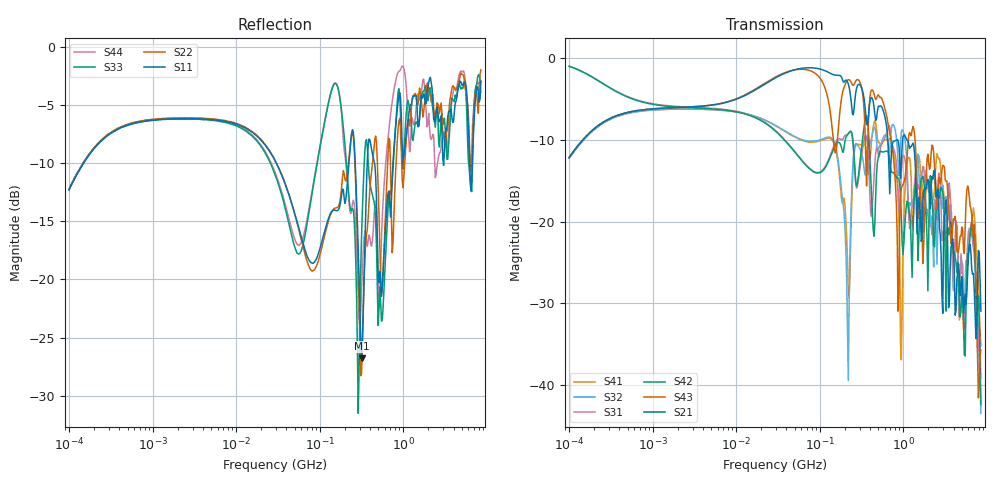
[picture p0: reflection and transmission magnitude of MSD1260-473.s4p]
# MHz S MA R 50
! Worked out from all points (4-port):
!   498 points, 100 kHz to 8.5 GHz, reference 50 ohm
!   strongest paths, dB at 100 kHz, 1.698 MHz, 29.49 MHz, 500.7 MHz, 8.5 GHz:
!     S21: -12.1, -6.1, -2.4, -6.0, -31.0
!     S43: -12.2, -6.1, -2.3, -4.5, -35.7
!     S42: -1.0, -5.9, -8.9, -12.2, -42.4
!     S31: -1.0, -5.9, -8.8, -11.6, -39.2
!     S32: -12.3, -6.2, -8.2, -11.3, -43.5
!     S41: -12.3, -6.2, -8.3, -10.3, -35.2
!   lowest |S11| = -26.8 dB at 317.1 MHz (marker M1), VSWR 1.10, Z = 54.1 - j2.43 ohm
!   |S11| at or under -10 dB: 30.11 MHz to 223.7 MHz (193.6 MHz wide, 153 % of centre); 452.9 MHz to 754.4 MHz (301.5 MHz wide, 49.9 % of centre); 6.23 GHz to 6.712 GHz (481.9 MHz wide, 7.45 % of centre)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
0.1  0.2423 59.0  0.2469 59.4  0.8944 -13.7  0.2436 -121.1
     0.2469 59.4  0.2444 58.9  0.2439 -121.2  0.8929 -13.8
     0.8944 -13.7  0.2439 -121.2  0.2428 58.9  0.2466 59.2
     0.2436 -121.1  0.8929 -13.8  0.2466 59.2  0.2443 58.9
136.2065  0.1935 0.7  0.8053 -32.8  0.2611 152.2  0.3205 8.9
          0.8053 -32.8  0.1915 3.6  0.3265 9.3  0.2542 155.0
          0.2611 152.2  0.3265 9.3  0.6335 -6.3  0.4361 -57.8
          0.3205 8.9  0.2542 155.0  0.4361 -57.8  0.6381 -5.2
220.0307  0.2934 -1.1  0.6961 -59.3  0.3446 39.0  0.0398 -109.0
          0.6961 -59.3  0.3109 -11.8  0.01064 -177.2  0.346 46.9
          0.3446 39.0  0.01064 -177.2  0.2436 -87.7  0.7395 -32.3
          0.0398 -109.0  0.346 46.9  0.7395 -32.3  0.2322 -79.7
317.0858  0.04589 -29.3  0.66 -70.8  0.2526 1.1  0.2958 11.4
          0.66 -70.8  0.03953 -19.7  0.2626 2.2  0.2831 10.5
          0.2526 1.1  0.2626 2.2  0.1539 15.2  0.6616 -78.9
          0.2958 11.4  0.2831 10.5  0.6616 -78.9  0.09095 -17.0
2110.57  0.7374 -176.2  0.1198 120.7  0.0943 69.0  0.1389 142.2
         0.1198 120.7  0.6191 -177.5  0.09367 98.1  0.1909 160.4
         0.0943 69.0  0.09367 98.1  0.6652 -177.4  0.2183 167.1
         0.1389 142.2  0.1909 160.4  0.2183 167.1  0.4068 173.6
6611.76  0.2669 90.8  0.05107 -5.3  0.08325 46.7  0.1011 95.3
         0.05107 -5.3  0.3062 64.7  0.09397 61.7  0.09845 73.8
         0.08325 46.7  0.09397 61.7  0.2382 69.9  0.1091 -40.6
         0.1011 95.3  0.09845 73.8  0.1091 -40.6  0.3699 66.1
8500  0.7098 -36.9  0.02824 -126.3  0.01099 -166.8  0.01731 -145.9
      0.02824 -126.3  0.7933 -45.9  0.006699 -155.1  0.007563 -116.8
      0.01099 -166.8  0.006699 -155.1  0.704 -54.1  0.01635 -14.3
      0.01731 -145.9  0.007563 -116.8  0.01635 -14.3  0.6354 -56.3
